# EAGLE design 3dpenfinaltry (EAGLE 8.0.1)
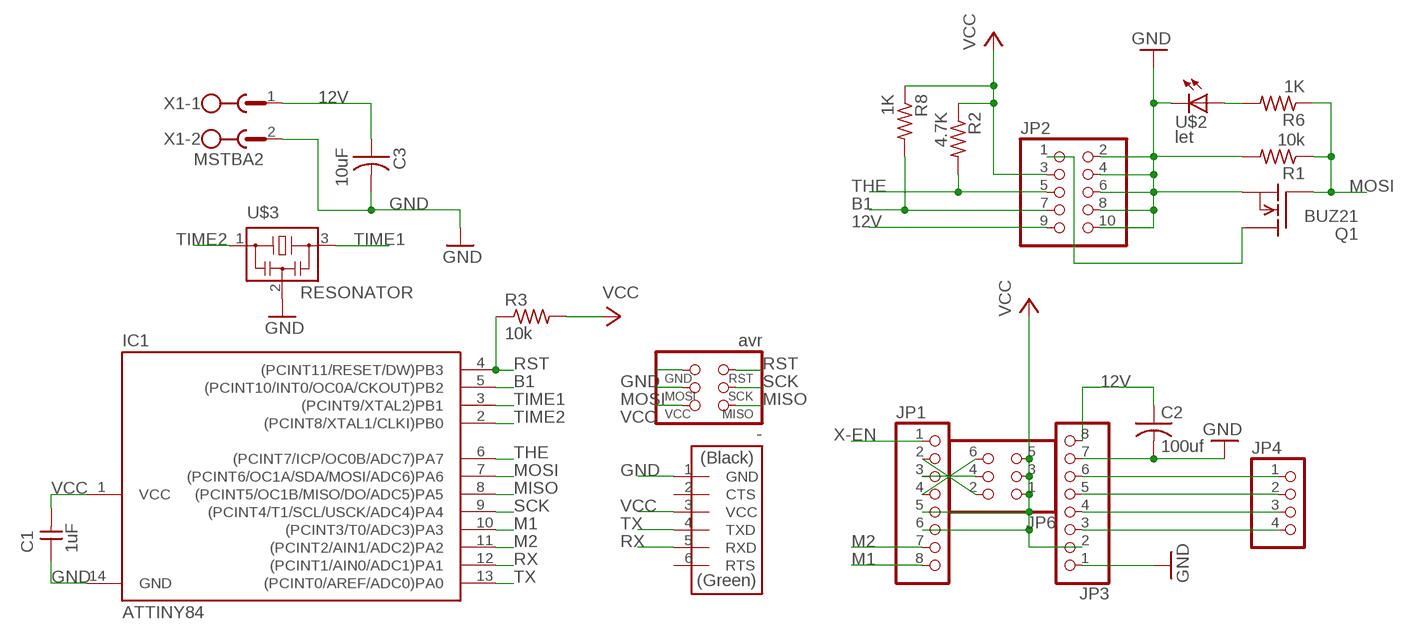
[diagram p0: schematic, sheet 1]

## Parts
-  avr  AVRISPSMD  [2X03SMD]
C1  1uF  CAP-UNPOLARIZEDFAB  [C1206FAB]
C2  100uf  C-US025-030X050  [C025-030X050]
C3  10uF  CAP-US1206FAB  [C1206FAB]
IC1  ATTINY84  ATTINY44-SSU  [SOIC14]
JP1  PINHD-1X8  [1X08]
JP2  PINHD-2X5  [2X05]
JP3  PINHD-1X8  [1X08]
JP4  PINHD-1X4  [1X04]
JP6  PINHD-2X3-SMD  [2X03SMD]
Q1  BUZ21  [TO220]
R1  10k  RES-US1206FAB  [R1206FAB]
R2  4.7K  RES-US1206FAB  [R1206FAB]
R3  10k  RES-US1206FAB  [R1206FAB]
R6  1K  RES-US1206FAB  [R1206FAB]
R8  1K  RES-US1206FAB  [R1206FAB]
U$1  FTDI-SMD-HEADER  [1X06SMD]
U$2  let  LEDFAB1206  [LED1206FAB]
U$3  RESONATOR  [EFOBM]
X1  MSTBA2  [MSTBA2]

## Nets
12V: C2.1 C3.1 JP2.9 JP3.8 X1.1
B1: IC1.5((PCINT10/INT0/OC0A/CKOUT)PB2) JP2.7 R8.2
GND: -.6(GND) C1.1 C2.2 C3.2 IC1.14(GND) JP2.2 JP2.4 JP2.6 JP2.8 JP2.10 JP3.1 JP3.7 Q1.3(S) R1.2 U$1.1(GND) U$2.2(C) U$3.2 X1.2
M1: IC1.10((PCINT3/T0/ADC3)PA3) JP1.8
M2: IC1.11((PCINT2/AIN1/ADC2)PA2) JP1.7
MISO: -.1(MISO) IC1.8((PCINT5/OC1B/MISO/DO/ADC5)PA5)
MOSI: -.4(MOSI) IC1.7((PCINT6/OC1A/SDA/MOSI/ADC6)PA6) Q1.1(G) R1.1 R6.1
N$1: JP2.1 Q1.2(D)
N$2: R6.2 U$2.1(A)
N$3: JP1.4 JP6.6
N$4: JP3.3 JP4.4
N$5: JP3.4 JP4.3
N$6: JP1.2 JP6.2
N$7: JP1.3 JP6.4
N$8: JP3.5 JP4.2
N$9: JP3.6 JP4.1
RST: -.5(RST) IC1.4((PCINT11/RESET/DW)PB3) R3.1
RX: IC1.12((PCINT1/AIN0/ADC1)PA1) U$1.5(RXD)
SCK: -.3(SCK) IC1.9((PCINT4/T1/SCL/USCK/ADC4)PA4)
THE: IC1.6((PCINT7/ICP/OC0B/ADC7)PA7) JP2.5 R2.2
TIME1: IC1.3((PCINT9/XTAL2)PB1) U$3.3
TIME2: IC1.2((PCINT8/XTAL1/CLKI)PB0) U$3.1
TX: IC1.13((PCINT0/AREF/ADC0)PA0) U$1.4(TXD)
VCC: -.2(VCC) C1.2 IC1.1(VCC) JP1.5 JP1.6 JP2.3 JP3.2 JP6.1 JP6.3 JP6.5 R2.1 R3.2 R8.1 U$1.3(VCC)
X-EN: JP1.1
Unconnected: U$1.2(CTS) U$1.6(RTS)

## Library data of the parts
- = fab:AVRISP
C1 = fab:CAP-UNPOLARIZED
C2 = rcl:C-US: CAPACITOR, American symbol
C3 = fab:CAP-US
IC1 = fab:ATTINY44
JP1 JP3 = pinhead:PINHD-1X8: PIN HEADER
JP2 = pinhead:PINHD-2X5: PIN HEADER
JP4 = pinhead:PINHD-1X4: PIN HEADER
JP6 = fab:PINHD-2X3-SMD: PIN HEADER
Q1 = transistor-fet:BUZ21: N-Channel Enhancement MOSFET 100V; 19A; 0,1Ohm
R1-R3 R6 R8 = fab:RES-US: Resistor (US Symbol)
U$1 = fab:FTDI-SMD-HEADER
U$2 = fab:LED: LED
U$3 = fab:RESONATOR
X1 = con-phoenix-508:MSTBA2: PHOENIX; MF: FARNELL; MPN: 1757242; OC_FARNELL: 3705171; OC_NEWARK: 71C4161

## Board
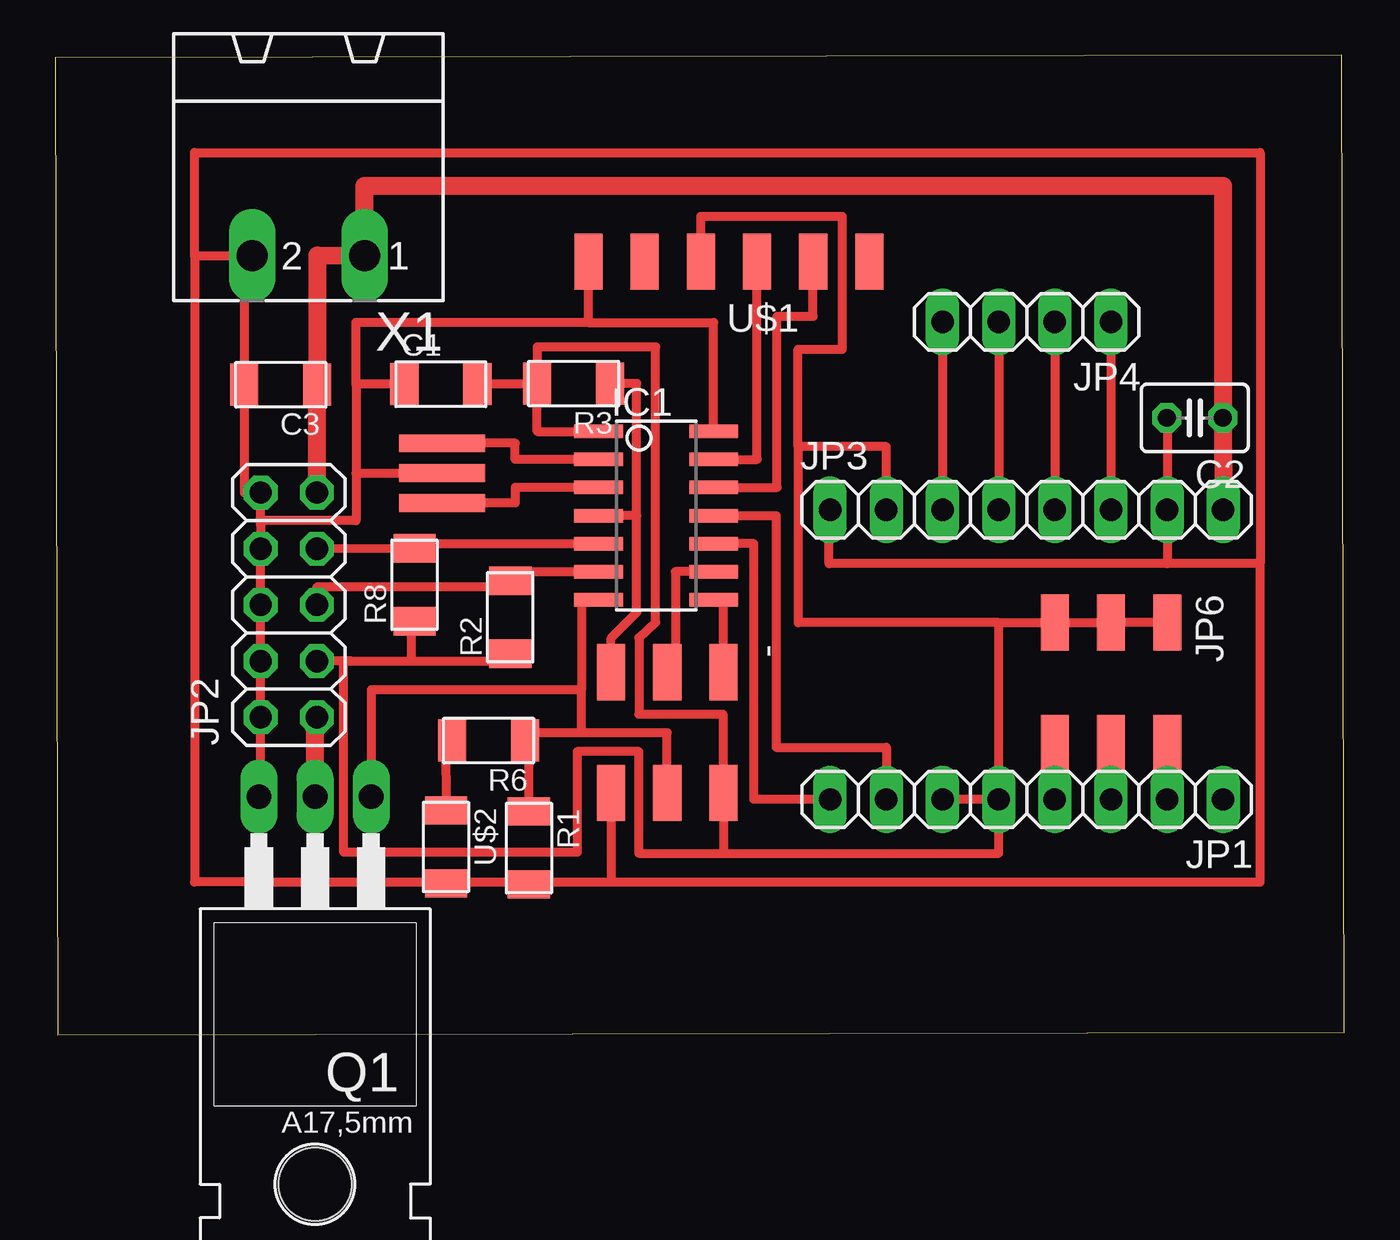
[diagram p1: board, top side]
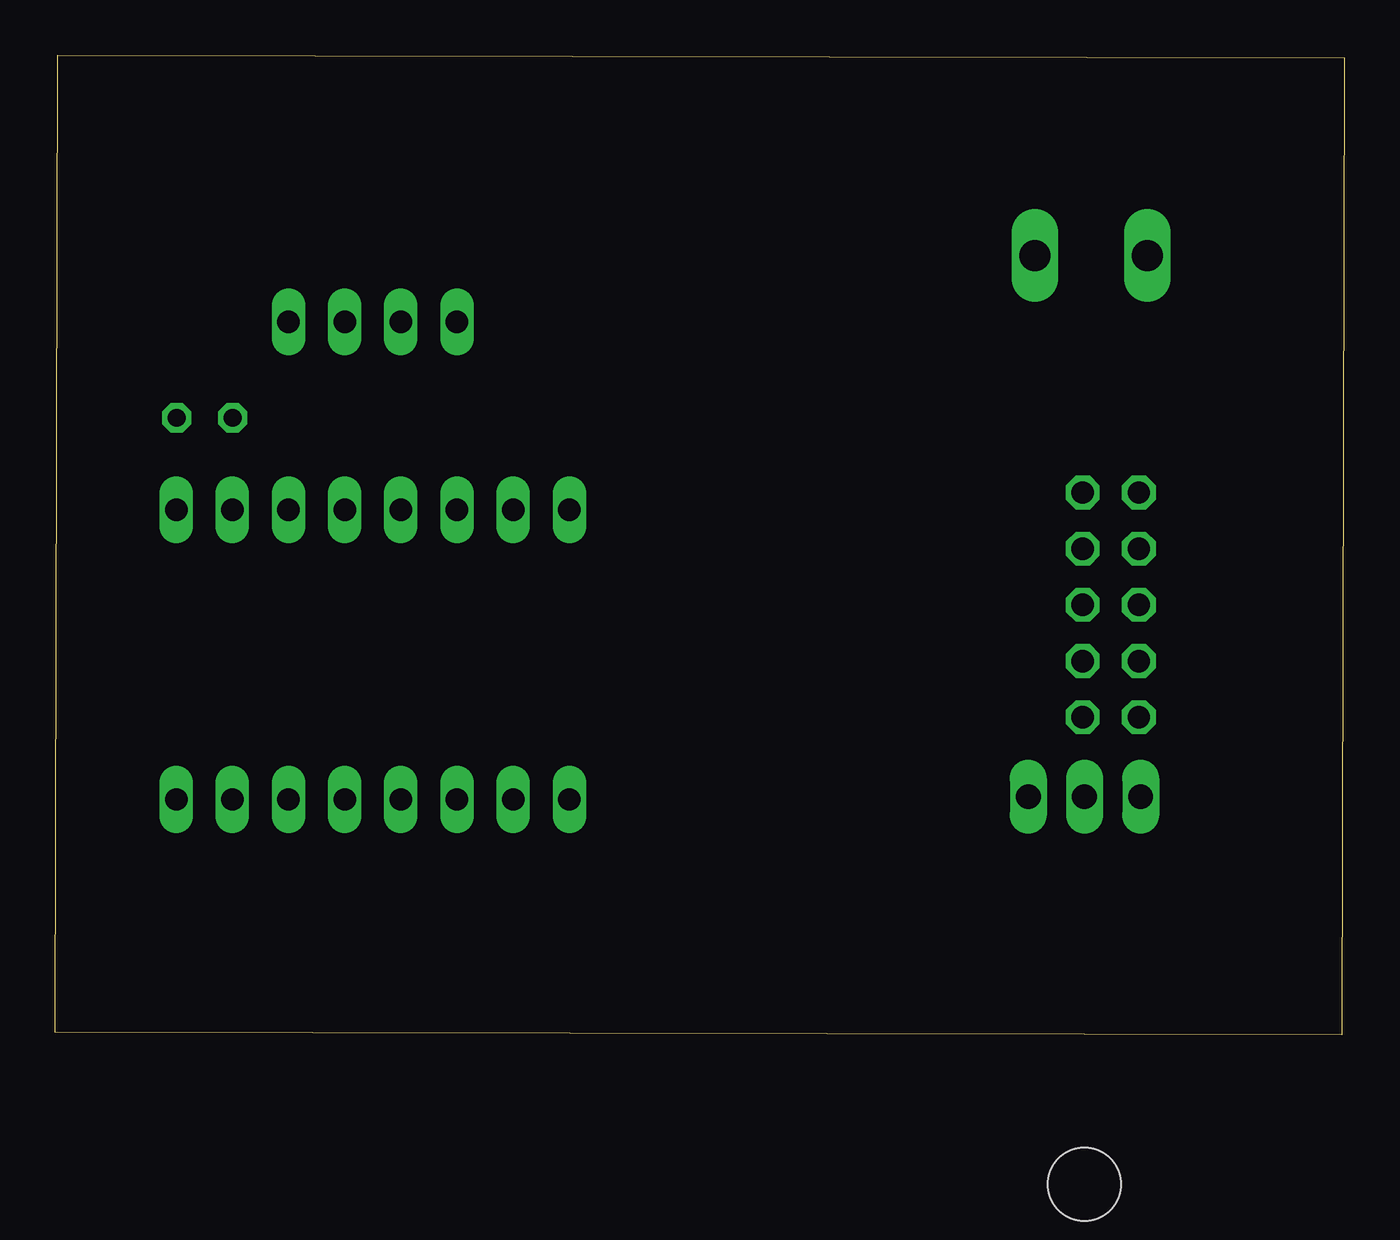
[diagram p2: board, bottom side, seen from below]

Size 58.3 x 44.3 mm. Coordinates in mm from the lower left corner, seen from the top.
Outline: 0.1,0 58.3,0.1 58.2,44.3 0,44.2 0.1,0
Copper layers (1*16): Top 0.035mm / dielectric 1.5mm / Bottom 0.035mm
Design rules "default *": minimum track width 10mil, minimum drill 24mil, track to track 16mil, track to pad 16mil, pad to pad 16mil, via to via 16mil, smd to smd 16mil, copper to edge 40mil, drill to drill 16mil, minimum pad ring 10mil, minimum via ring 8mil, stop-mask expansion 4mil, vias tented up to drill 0mil, thermal gap 10mil

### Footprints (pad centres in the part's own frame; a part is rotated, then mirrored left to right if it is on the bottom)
2X03SMD = smd 2.54 x 1.27: 1 -2.54,2.54; 2 2.92,2.54; 3 -2.54,0; 4 2.92,0; 5 -2.54,-2.54; 6 2.92,-2.54
C1206FAB = smd 1.27 x 1.905: 1 -1.651,0; 2 1.651,0
C025-030X050 = drill 0.813 octagon: 1 -1.27,0; 2 1.27,0
SOIC14 = smd 0.61 x 2.21: 1 -3.81,-2.603; 2 -2.54,-2.603; 3 -1.27,-2.603; 4 0,-2.603; 5 1.27,-2.603; 6 2.54,-2.603; 7 3.81,-2.603; 8 3.81,2.603; 9 2.54,2.603; 10 1.27,2.603; 11 0,2.603; 12 -1.27,2.603; 13 -2.54,2.603; 14 -3.81,2.603
1X08 = drill 1.016 long: 1 -8.89,0; 2 -6.35,0; 3 -3.81,0; 4 -1.27,0; 5 1.27,0; 6 3.81,0; 7 6.35,0; 8 8.89,0
2X05 = drill 1.016 octagon: 1 -5.08,-1.27; 2 -5.08,1.27; 3 -2.54,-1.27; 4 -2.54,1.27; 5 0,-1.27; 6 0,1.27; 7 2.54,-1.27; 8 2.54,1.27; 9 5.08,-1.27; 10 5.08,1.27
1X04 = drill 1.016 long: 1 -3.81,0; 2 -1.27,0; 3 1.27,0; 4 3.81,0
TO220 = drill 1.118 long: 1 -2.54,-6.35; 2 0,-6.35; 3 2.54,-6.35 | hole 3.302: 0,11.176
R1206FAB = smd 1.27 x 1.905: 1 -1.651,0; 2 1.651,0
1X06SMD = smd 2.54 x 1.27: 1 0,6.35; 2 0,3.81; 3 0,1.27; 4 0,-1.27; 5 0,-3.81; 6 0,-6.35
LED1206FAB = smd 1.27 x 1.905: 1 -1.651,0; 2 1.651,0
EFOBM = smd 0.8 x 3.9: 1 -1.35,0; 2 0,0; 3 1.35,0
MSTBA2 = drill 1.397 long: 1 -2.54,5.08; 2 2.54,5.08

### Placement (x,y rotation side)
-  27.68,13.85 270 top
C1  17.44,29.42 0 top
C2  51.54,27.9 180 top
C3  10.2,29.4 180 top
IC1  27.18,23.48 270 top
JP1  43.94,10.64 180 top
JP2  10.56,19.44 90 top
JP3  43.94,23.74 0 top
JP4  43.94,32.24 180 top
JP6  47.75,16.1 270 top
Q1  11.75,4.41 180 top
R1  21.42,8.44 270 top
R2  20.58,18.88 90 top
R3  23.45,29.45 180 top
R6  19.6,13.3 180 top
R8  16.25,20.35 90 top
U$1  30.47,34.97 90 top
U$2  17.67,8.49 270 top
U$3  17.5,25.4 270 top
X1  11.45,40.32 180 top

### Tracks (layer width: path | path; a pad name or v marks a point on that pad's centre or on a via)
12V
  Top 0.813: JP2.9 11.83,27.6 C3.1 11.85,35.25 X1.1 13.99,38.4 52.81,38.4 C2.1 JP3.8
B1
  Top 0.406: 16.2,22.21 IC1.5 | 16.2,22.21 15.7,22.21 | JP2.7 R8.2 16.2,21.95 16.2,22.21
GND
  Top 0.406: 21.4,6.9 25.14,6.9 | 17.5,6.9 21.4,6.9 | 9.4,6.9 17.5,6.9 | 9.4,6.9 6.3,6.9 6.3,35.24 | 6.3,35.24 6.3,39.9 54.5,39.9 54.5,21.3 | 13.6,25.4 U$3.2 | 13.6,25.4 13.6,23.25 9.29,23.25 9.29,23 | -.6 25.14,6.9 | IC1.14 29.78,32.21 24.1,32.21 | 24.18,35.43 U$1.1 24.1,34.87 24.1,32.21 | 24.1,32.21 13.6,32.21 13.6,29.42 | 13.6,29.42 13.6,25.4 | C1.1 13.6,29.42 | 6.3,35.24 X1.2 8.55,35.24 C3.2 8.55,24.52 JP2.10 9.29,23 | R1.2 21.4,6.9 | U$2.2 17.5,6.9 | 50.29,21.3 JP3.7 50.29,27.9 C2.2 | 50.29,21.3 35,21.3 35,23.74 JP3.1 | 54.5,21.3 50.29,21.3 | 25.14,6.9 54.5,6.9 54.5,21.3 | 9.29,23 JP2.8 JP2.6 JP2.4 JP2.2 9.29,10.76 Q1.3 9.21,6.9 9.4,6.9
  Bottom 0.406: JP3.7 50.27,23.74
M1
  Top 0.406: JP1.8 31.6,10.64 31.6,22.21 IC1.10
M2
  Top 0.406: IC1.11 32.6,23.48 32.6,13 37.59,13 JP1.7
MISO
  Top 0.406: -.1 30.23,19.69 IC1.8
MOSI
  Top 0.406: IC1.7 23.8,19.67 23.8,15.6 | 23.8,13.65 23.8,15.6 | 21.42,13.65 R6.1 | R1.1 21.42,13.65 | 23.8,15.6 14.29,15.6 Q1.1 | 27.38,11.02 -.4 27.68,13.65 23.8,13.65 | 23.8,13.65 21.42,13.65
N$1
  Top 0.813: Q1.2 11.75,14.36 JP2.1
N$2
  Top 0.406: R6.2 17.65,13.34 U$2.1
N$3
  Top 0.406: JP6.6 JP1.4
N$4
  Top 0.406: JP4.4 JP3.3
N$5
  Top 0.406: JP4.3 JP3.4
N$6
  Top 0.406: JP6.2 JP1.2
N$7
  Top 0.406: JP6.4 JP1.3
N$8
  Top 0.406: JP4.2 JP3.5
N$9
  Top 0.406: JP4.1 JP3.6
RST
  Top 0.406: 26.3,23.48 IC1.4 | 26.3,23.48 26.3,29.45 R3.1 | 25.1,16.39 -.5 25.14,17.94 26.3,19.1 26.3,23.48
RX
  Top 0.406: IC1.12 32.65,24.75 32.65,32.5 34.28,32.5 U$1.5
SCK
  Top 0.406: IC1.9 28.05,20.94 28.05,17.39 -.3
THE
  Top 0.406: IC1.6 21.38,20.94 20.58,20.93 R2.2 20.29,20.53 20.29,20.24 11.83,20.24 JP2.5
TIME1
  Top 0.406: IC1.3 20.8,24.75 20.8,24.05 U$3.3
TIME2
  Top 0.406: IC1.2 20.8,26.02 20.8,26.75 U$3.1
TX
  Top 0.406: IC1.13 31.74,26.02 U$1.4
VCC
  Top 0.406: IC1.1 21.8,27.29 21.8,29.42 | U$1.3 29.2,37 35.6,37 35.6,31 33.6,31 33.6,26.6 | 21.8,29.42 R3.2 21.8,29.25 21.8,31.1 27.15,31.1 27.15,18.65 26.4,17.95 26.4,14.5 30.2,14.5 30.2,10.93 -.2 30.22,8.2 | 21.8,29.42 C1.2 | R2.1 20.25,16.9 16.1,16.9 | 13.4,16.9 JP2.3 | 13.4,16.9 16.1,16.9 | R8.1 16.1,18.5 16.1,16.9 | JP6.1 JP6.3 JP6.5 42.67,18.64 | JP1.5 JP1.6 | 42.67,18.64 33.6,18.64 33.6,26.6 | JP3.2 37.59,26.6 33.6,26.6 | 30.22,8.2 26.4,8.2 26.4,12.8 23.6,12.8 23.6,8.25 13.05,8.25 13.05,16.9 13.4,16.9 | JP1.5 42.67,18.64 | 30.22,8.2 42.67,8.2 JP1.5
X-EN
  Top 0.406: JP1.1 52.8,10.64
